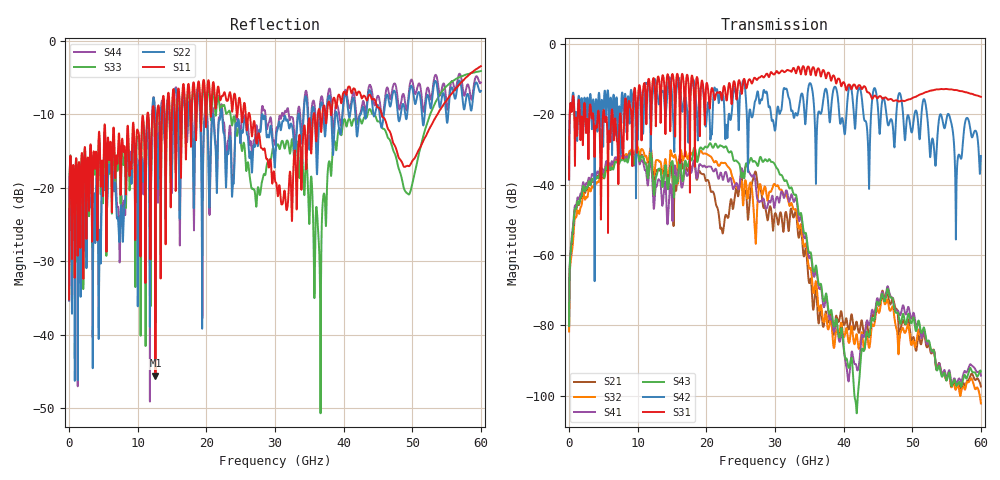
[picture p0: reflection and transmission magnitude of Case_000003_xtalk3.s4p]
! Info: Touchstone file created by circ.  Input file=CasetestDOE_NRZ_template_000003.circ
# Hz S RI R 50
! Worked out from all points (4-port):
!   6000 points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, 10 MHz to 60 GHz, reference 50 ohm
!   strongest paths, dB at 10 MHz, 15.01 GHz, 30.01 GHz, 45.01 GHz, 60 GHz:
!     S31: -38.4, -8.6, -8.4, -15.3, -15.0
!     S42: -38.6, -14.8, -24.6, -18.3, -31.8
!     S43: -80.1, -33.3, -34.3, -73.6, -93.1
!     S41: -79.5, -46.3, -45.5, -72.5, -94.3
!     S32: -81.7, -31.7, -40.0, -75.7, -102.2
!     S21: -80.3, -37.0, -48.1, -73.7, -97.4
!   lowest |S11| = -45.6 dB at 12.59 GHz (marker M1), VSWR 1.01, Z = 49.6 - j0.378 ohm
!   |S11| at or under -10 dB: start of sweep to 11.41 GHz; 26.31 GHz to 35.63 GHz (9.314 GHz wide, 30.1 % of centre); 45.55 GHz to 53.67 GHz (8.122 GHz wide, 16.4 % of centre)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
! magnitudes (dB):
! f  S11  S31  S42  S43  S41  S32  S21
! 10 MHz  -35.2  -38.4  -38.6  -80.1  -79.5  -81.7  -80.3
! 3.51 GHz  -16.0  -20.1  -15.8  -38.7  -37.4  -40.8  -39.2
! 12.59 GHz  -45.6  -18.8  -10.3  -38.8  -41.2  -33.9  -36.5
! 29.39 GHz  -16.4  -8.0  -19.5  -33.4  -44.7  -42.0  -46.5
! 36.53 GHz  -9.7  -7.9  -19.5  -68.6  -69.6  -75.7  -77.0
! 40.07 GHz  -6.9  -11.0  -24.6  -87.3  -87.6  -83.3  -79.9
! 60 GHz  -3.4  -15.0  -31.8  -93.1  -94.3  -102.2  -97.4
